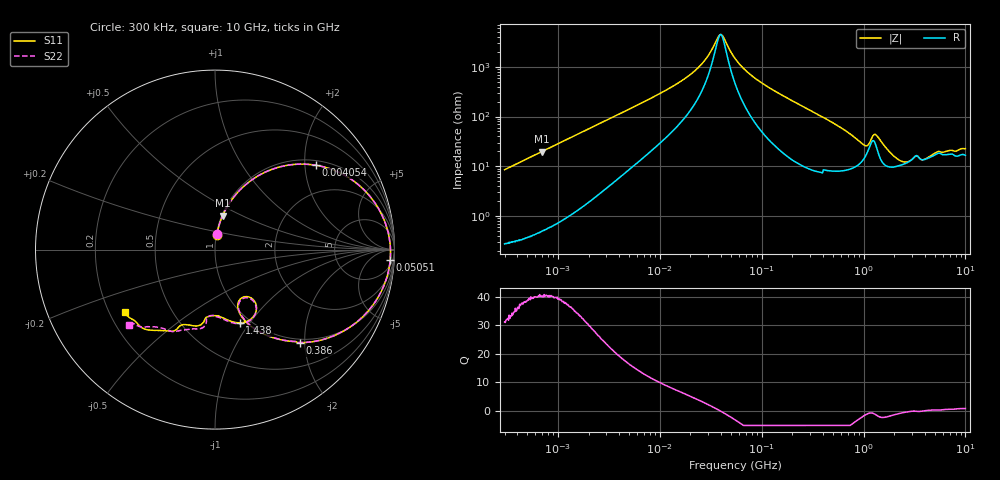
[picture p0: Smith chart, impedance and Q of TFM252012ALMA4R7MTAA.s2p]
! S-Parameter Data Generated by TDK Corporation
! Copyright(C) 2019 TDK Corporation.
! All Rights Reserved.
! TDK P/N: TFM252012ALMA4R7MTAA (Inductor)
! Property: L=4.7uH at 1MHz
! Size(LxWxT): 2.5x2x1.2mm
! Model Type: s2p (Touchstone File Format Version 1.0)
! Frequency: DC=Yes Start=0.3MHz Stop=10000MHz 802points Log-sweep
! Model Generated on May 10, 2019
! Port Assignments:
!  1 ---@@@--- 2
! Applicable Conditions:
!  Temperature = 25 degC
!  DC Bias Current = 0 A
!  Small Signal Operation
! Terms and conditions regarding TDK Simulation Models
! (1)This simulation model is being provided solely for informational purposes. Please refer to the specifications of the products in terms of detailed characteristics of such products.
! (2)In no event shall TDK Corporation of any of its subsidiaries be liable for any loss or damage arising, directly or indirectly,
!  From any information contained in this simulation model, including, but not limited to loss or damages arising from any inaccuracies, omissions or errors in connection with such information.
! (3)Any and all copyrights on this simulation model are owned by TDK Corporation.
!  Duplication or redistribution of this simulation model without prior written permission from TDK Corporation is prohibited.
! (4)This simulation model is subject to any modification or change without any prior notice.
! (5)Neither TDK Corporation nor any of its subsidiaries shall make any warranty, express or implied,
!  Including but not limited to the correctness, implied warranties of merchantability and fitness for a particular purpose with respect to this simulation models.
! (6)The use of this simulation model shall be deemed to have consented to the terms and conditions hereof.
# Hz S MA R 50
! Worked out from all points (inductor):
!   801 points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, 300 kHz to 10 GHz, reference 50 ohm
!   read as one part in series: L = 4.51 uH near 318.3 kHz
!   highest Q = 40.3 at 698.2 kHz (marker M1), where L = 4.51 uH
!   self-resonance near 39.57 MHz
!   S11 on the Smith chart (normalised r, x): 300 kHz: 1.01, +0.17; 4.054 MHz: 1.12, +2.28; 50.51 MHz: 11, -29; 386 MHz: 0.93, -1.90; 1.438 GHz: 0.90, -0.90; 10 GHz: 0.26, -0.29
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300000  0.08452 83.4  0.9937 -4.9  0.9935 -4.9  0.08483 83.4
698226  0.193 77.4  0.9765 -11.1  0.9762 -11.1  0.193 77.4
1713600  0.4299 62.8  0.8899 -25.5  0.8897 -25.5  0.4299 62.8
4053600  0.7324 39.9  0.6435 -47.1  0.6435 -47.1  0.7325 39.9
9671944  0.9134 18.9  0.3277 -65.5  0.3277 -65.5  0.9134 18.9
2.346945e7  0.97 5.4  0.1042 -70.7  0.1042 -70.7  0.97 5.4
2.987769e7  0.9752 2.6  0.0582 -63.8  0.05821 -63.8  0.9752 2.6
3.86086e7  0.978 -0.3  0.02247 -12.2  0.02246 -12.3  0.978 -0.3
4.199124e7  0.9783 -1.3  0.02436 26.2  0.02438 26.2  0.9783 -1.3
5.051192e7  0.9779 -3.5  0.05131 62.4  0.05132 62.4  0.9779 -3.5
5.477226e7  0.9772 -4.5  0.0662 67.2  0.06621 67.2  0.9772 -4.5
1.063884e8  0.9551 -14.2  0.2174 70.3  0.2175 70.3  0.9551 -14.1
3.126428e8  0.7726 -40.9  0.5876 45.5  0.5875 45.5  0.7728 -40.8
3.860116e8  0.7026 -47.6  0.6636 38.4  0.6636 38.4  0.7029 -47.4
7.400828e8  0.4508 -66.2  0.8204 14.9  0.8204 14.9  0.451 -65.9
1.069912e9  0.3105 -63.4  0.8135 -0.7  0.8135 -0.7  0.3161 -63.1
1.260284e9  0.4002 -54.6  0.7059 -0.9  0.7058 -0.9  0.4071 -55.6
1.43752e9  0.4307 -71.3  0.7819 1.5  0.7818 1.5  0.4336 -72.3
1.767019e9  0.3831 -83.3  0.8375 -6.7  0.8374 -6.7  0.3845 -84.7
4.632637e9  0.4588 -113.8  0.7313 -42.4  0.7312 -42.4  0.4746 -109.7
7.141296e9  0.5658 -127.3  0.6199 -63.0  0.6199 -63.0  0.5639 -130.2
1e10  0.6117 -145.1  0.538 -80.1  0.5382 -80.1  0.6361 -138.6
